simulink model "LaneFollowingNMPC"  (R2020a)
settings: Solver=FixedStepAuto  StartTime=0.0  StopTime=Duration  FixedStep=0.1  RelTol=1e-3  EnableMultiTasking=on
PreLoadFcn:
  | LaneFollowingUsingNMPCData
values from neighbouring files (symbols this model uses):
  Cf = 19000    [LaneFollowingStateFcn.m]    (also in LaneFollowingUsingNMPCData.m)
  Cr = 33000    [LaneFollowingStateFcn.m]    (also in LaneFollowingUsingNMPCData.m)
  Iz = 2875    [LaneFollowingStateFcn.m]    (also in LaneFollowingUsingNMPCData.m)
  lf = 1.2    [LaneFollowingStateFcn.m]    (also in LaneFollowingUsingNMPCData.m)
  lr = 1.6    [LaneFollowingStateFcn.m]    (also in LaneFollowingUsingNMPCData.m)
  m = 1575    [LaneFollowingStateFcn.m]    (also in LaneFollowingUsingNMPCData.m)
  rho = LaneFollowingGetCurvature(v_set,t)    [LaneFollowingUsingNMPCData.m]
  tau = 0.2    [LaneFollowingStateFcn.m]    (also in LaneFollowingUsingNMPCData.m)
  Ts = u(5)    [LaneFollowingEKFStateFcn.m]    (also in LaneFollowingUsingNMPCData.m = 0.1)
  v0 = 15    [LaneFollowingUsingNMPCData.m]
  v_set = 20    [LaneFollowingUsingNMPCData.m]
libraries: sharedTrackingLibrary x1, mpclib x1

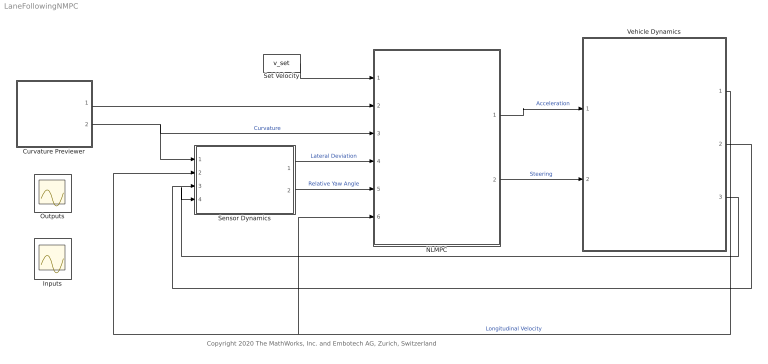
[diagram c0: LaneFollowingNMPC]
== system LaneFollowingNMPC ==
  note: Copyright 2020 The MathWorks, Inc. and Embotech AG, Zurich, Switzerland
  Curvature Previewer : Subsystem  mask{signal=rho, ts=Ts, steps=10}
      mask prompts: signal "Signal name"; ts "Sampling time"; steps "Number of previewing steps"
      mask init:
      | ts = evalin('base',get_param(gcbh,'ts'));
      | signal = evalin('base',get_param(gcbh,'signal'));
      | steps = evalin('base',get_param(gcbh,'steps'));
      | data = mpc_previewer_maskinit(signal,ts);
  Inputs : Scope
  NLMPC : Subsystem  VariantControl=controller_type ==1
  Outputs : Scope
  Sensor Dynamics : Subsystem
  Set Velocity : Constant  Value=v_set
  Vehicle Dynamics : Subsystem
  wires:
  Curvature Previewer/2(current) -> NLMPC/3(Current Curvature), Sensor Dynamics/1(Current curvature)  "Curvature"
  Vehicle Dynamics/2(Lateral Velocity) -> Sensor Dynamics/3(Lateral velocity)
  Vehicle Dynamics/3(Yaw Rate) -> Sensor Dynamics/4(Yaw rate)
  Vehicle Dynamics/1(Longitudinal Velocity) -> NLMPC/6(Longitudinal Velocity), Sensor Dynamics/2(Longitudinal velocity)  "Longitudinal Velocity"
  Curvature Previewer/1(sequence) -> NLMPC/2(Curvature Sequence)
  Sensor Dynamics/1(Lateral deviation) -> NLMPC/4(Lateral Deviation)  "Lateral Deviation"
  Sensor Dynamics/2(Relative yaw angle) -> NLMPC/5(Relative Yaw Angle)  "Relative Yaw Angle"
  Set Velocity/1 -> NLMPC/1(Set velocity)
  NLMPC/1(Acceleration) -> Vehicle Dynamics/1(Acceleration)  "Acceleration"
  NLMPC/2(Steering) -> Vehicle Dynamics/2(Steering)  "Steering"

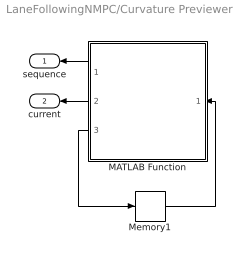
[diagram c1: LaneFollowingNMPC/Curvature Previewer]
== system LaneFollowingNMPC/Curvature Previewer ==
  MATLAB Function : MATLAB Function  TreatAsAtomicUnit=on
  Memory1 : Memory  InheritSampleTime=on  LinearizeAsDelay=on
  sequence : Outport  VectorParamsAs1DForOutWhenUnconnected=off
  current : Outport  Port=2  VectorParamsAs1DForOutWhenUnconnected=off
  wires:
  MATLAB Function/1(seq) -> sequence/1
  MATLAB Function/2(first) -> current/1
  Memory1/1 -> MATLAB Function/1(t)
  MATLAB Function/3(next_t) -> Memory1/1

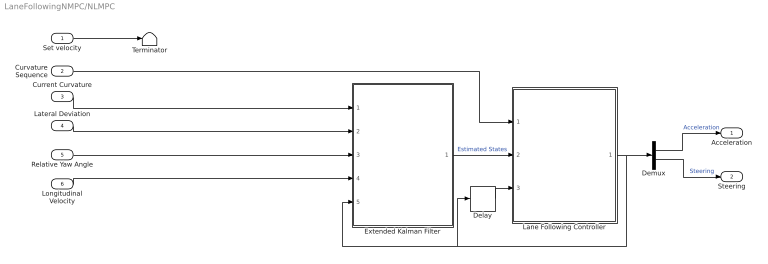
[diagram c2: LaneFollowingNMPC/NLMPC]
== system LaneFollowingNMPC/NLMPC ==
  Set velocity : Inport
  Curvature Sequence : Inport  Port=2
  Current Curvature : Inport  Port=3
  Lateral Deviation : Inport  Port=4
  Relative Yaw Angle : Inport  Port=5
  Longitudinal Velocity : Inport  Port=6
  Delay : Delay  DelayLength=1  InitialCondition=[0.2 0.3]
  Demux : Demux  Outputs=2
  Extended Kalman Filter : Subsystem
  Lane Following Controller : Subsystem
  Terminator : Terminator
  Acceleration : Outport  VectorParamsAs1DForOutWhenUnconnected=off
  Steering : Outport  Port=2  VectorParamsAs1DForOutWhenUnconnected=off
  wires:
  Extended Kalman Filter/1(xhat) -> Lane Following Controller/2(Estimated States)  "Estimated States"
  Lane Following Controller/1(Current MVs) -> Demux/1, Extended Kalman Filter/5(MVs), Delay/1
  Lateral Deviation/1 -> Extended Kalman Filter/2(Lateral Deviation)
  Curvature Sequence/1 -> Lane Following Controller/1(Curvature Sequence)
  Longitudinal Velocity/1 -> Extended Kalman Filter/4(Longitudinal Velocity)
  Delay/1 -> Lane Following Controller/3(Previous MVs)
  Relative Yaw Angle/1 -> Extended Kalman Filter/3(Relative Yaw Angle)
  Current Curvature/1 -> Extended Kalman Filter/1(Current Curvature)
  Set velocity/1 -> Terminator/1
  Demux/2 -> Steering/1  "Steering"
  Demux/1 -> Acceleration/1  "Acceleration"

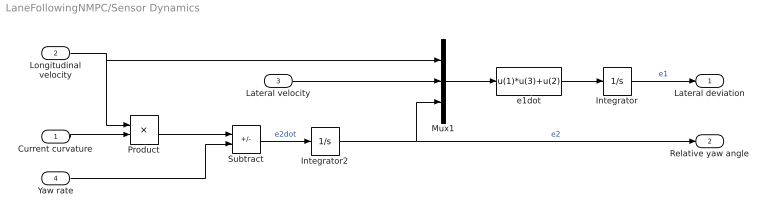
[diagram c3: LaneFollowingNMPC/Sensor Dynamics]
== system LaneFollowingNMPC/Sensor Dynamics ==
  Current curvature : Inport
  Longitudinal velocity : Inport  Port=2
  Lateral velocity : Inport  Port=3
  Yaw rate : Inport  Port=4
  Integrator : Integrator
  Integrator2 : Integrator
  Mux1 : Mux  Inputs=[1 1 1]
  Product : Product
  Subtract : Sum  Inputs=-+
  e1dot : Fcn  Expr=u(1)*u(3)+u(2)
  Lateral deviation : Outport  VectorParamsAs1DForOutWhenUnconnected=off
  Relative yaw angle : Outport  Port=2  VectorParamsAs1DForOutWhenUnconnected=off
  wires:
  Current curvature/1 -> Product/2
  Mux1/1 -> e1dot/1
  e1dot/1 -> Integrator/1
  Longitudinal velocity/1 -> Product/1, Mux1/1
  Lateral velocity/1 -> Mux1/2
  Integrator/1 -> Lateral deviation/1  "e1"
  Product/1 -> Subtract/1
  Yaw rate/1 -> Subtract/2
  Subtract/1 -> Integrator2/1  "e2dot"
  Integrator2/1 -> Mux1/3, Relative yaw angle/1  "e2"

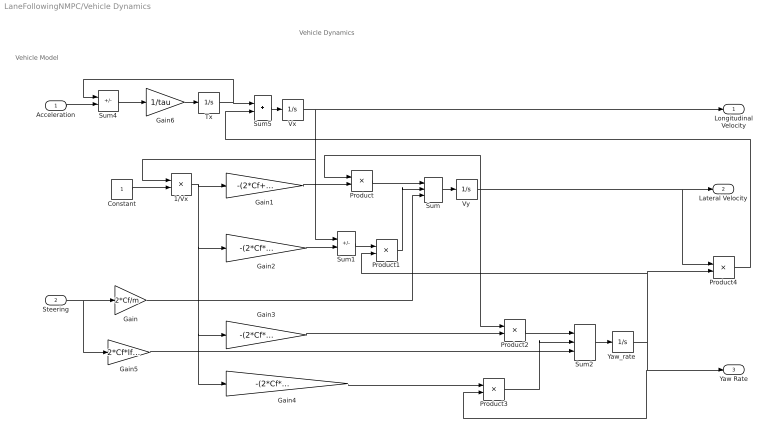
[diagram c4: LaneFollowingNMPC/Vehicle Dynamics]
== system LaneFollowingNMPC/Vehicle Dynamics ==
  note: Vehicle Model
  note: Vehicle Dynamics
  Acceleration : Inport
  Steering : Inport  Port=2
  1/Vx : Product  Inputs=/*
  Constant : Constant
  Gain : Gain  Gain=2*Cf/m
  Gain1 : Gain  Gain=-(2*Cf+2*Cr)/m
  Gain2 : Gain  Gain=-(2*Cf*lf-2*Cr*lr)/m
  Gain3 : Gain  Gain=-(2*Cf*lf-2*Cr*lr)/Iz
  Gain4 : Gain  Gain=-(2*Cf*lf^2+2*Cr*lr^2)/Iz
  Gain5 : Gain  Gain=2*Cf*lf/Iz
  Gain6 : Gain  Gain=1/tau
  Product{,1..4} (5 alike) : Product
  Sum : Sum  Inputs=+++
  Sum1 : Sum  Inputs=-+
  Sum2 : Sum  Inputs=+++
  Sum4 : Sum  Inputs=-+
  Sum5 : Sum
  Tx : Integrator
  Vx : Integrator  InitialCondition=v0
  Vy : Integrator
  "Yaw_rate " : Integrator
  Longitudinal Velocity : Outport  VectorParamsAs1DForOutWhenUnconnected=off
  Lateral Velocity : Outport  Port=2  VectorParamsAs1DForOutWhenUnconnected=off
  Yaw Rate : Outport  Port=3  VectorParamsAs1DForOutWhenUnconnected=off
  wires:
  Gain6/1 -> Tx/1
  Sum2/1 -> "Yaw_rate "/1
  Sum5/1 -> Vx/1
  Gain2/1 -> Sum1/2
  Gain4/1 -> Product3/1
  Constant/1 -> 1/Vx/2
  Gain3/1 -> Product2/2
  1/Vx/1 -> Gain4/1, Gain3/1, Gain2/1, Gain1/1
  Product2/1 -> Sum2/1
  Sum4/1 -> Gain6/1
  Acceleration/1 -> Sum4/2
  Tx/1 -> Sum5/1, Sum4/1
  Product3/1 -> Sum2/2
  Gain5/1 -> Sum2/3
  Product4/1 -> Sum5/2
  Sum1/1 -> Product1/1
  "Yaw_rate "/1 -> Yaw Rate/1, Product3/2, Product4/2, Product1/2
  Gain/1 -> Sum/3
  Steering/1 -> Gain/1, Gain5/1
  Gain1/1 -> Product/2
  Product/1 -> Sum/1
  Vy/1 -> Product/1, Lateral Velocity/1, Product4/1, Product2/1
  Sum/1 -> Vy/1
  Vx/1 -> Longitudinal Velocity/1, 1/Vx/1, Sum1/1
  Product1/1 -> Sum/2

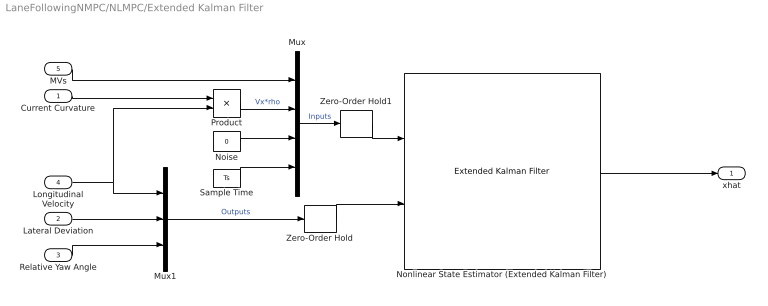
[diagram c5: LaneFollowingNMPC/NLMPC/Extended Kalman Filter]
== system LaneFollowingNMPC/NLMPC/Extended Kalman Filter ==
  Current Curvature : Inport
  Lateral Deviation : Inport  Port=2
  Relative Yaw Angle : Inport  Port=3
  Longitudinal Velocity : Inport  Port=4
  MVs : Inport  Port=5
  Mux : Mux
  Mux1 : Mux  Inputs=3
  Noise : Constant  Value=0
  Nonlinear State Estimator (Extended Kalman Filter) : sharedTrackingLibrary/Extended Kalman Filter  StateTransitionFcn=LaneFollowingEKFStateFcn  HasStateTransitionJacobianFcn=off  HasAdditiveProcessNoise=Additive  ProcessNoise=1e-4*eye(7)  HasTimeVaryingProcessNoise=off  HasStateTransitionFcnExtraArgument=1  InitialState=[0 0 v0 0 0 0 0]'  InitialStateCovariance=1e-4*eye(7)  MeasurementFcn1=LaneFollowingEKFMeasFcn  HasMeasurementJacobianFcn1=off  HasMeasurementEnablePort1=off  HasAdditiveMeasurementNoise1=Additive  MeasurementNoise1=1e-4*eye(3)  HasTimeVaryingMeasurementNoise1=off  HasMeasurementFcnExtraArgument1=0  MeasurementFcn2=myMeasurementFcn  HasMeasurementJacobianFcn2=off  HasMeasurementEnablePort2=off  HasAdditiveMeasurementNoise2=Additive  MeasurementNoise2=1  HasTimeVaryingMeasurementNoise2=off  HasMeasurementFcnExtraArgument2=0  MeasurementFcn3=myMeasurementFcn  HasMeasurementJacobianFcn3=off  HasMeasurementEnablePort3=off  HasAdditiveMeasurementNoise3=Additive  MeasurementNoise3=1  HasTimeVaryingMeasurementNoise3=off  HasMeasurementFcnExtraArgument3=0  MeasurementFcn4=myMeasurementFcn  HasMeasurementJacobianFcn4=off  HasMeasurementEnablePort4=off  HasAdditiveMeasurementNoise4=Additive  MeasurementNoise4=1  HasTimeVaryingMeasurementNoise4=off  HasMeasurementFcnExtraArgument4=0  MeasurementFcn5=myMeasurementFcn  HasMeasurementJacobianFcn5=off  HasMeasurementEnablePort5=off  HasAdditiveMeasurementNoise5=Additive  MeasurementNoise5=1  HasTimeVaryingMeasurementNoise5=off  HasMeasurementFcnExtraArgument5=0  EnableMultirate=off  StateTransitionFcnSampleTime=1  MeasurementFcn1SampleTime=1  MeasurementFcn2SampleTime=1  MeasurementFcn3SampleTime=1  MeasurementFcn4SampleTime=1  MeasurementFcn5SampleTime=1  UseCurrentEstimator=on  OutputStateCovariance=off  DataType=double  SampleTime=Ts  NumberOfMeasurements=1
  Product : Product
  Sample Time : Constant  Value=Ts
  Zero-Order Hold : ZeroOrderHold  SampleTime=Ts
  Zero-Order Hold1 : ZeroOrderHold  SampleTime=Ts
  xhat : Outport  VectorParamsAs1DForOutWhenUnconnected=off
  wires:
  Noise/1 -> Mux/3
  Zero-Order Hold/1 -> Nonlinear State Estimator (Extended Kalman Filter)/2
  MVs/1 -> Mux/1
  Sample Time/1 -> Mux/4
  Nonlinear State Estimator (Extended Kalman Filter)/1 -> xhat/1
  Mux1/1 -> Zero-Order Hold/1  "Outputs"
  Lateral Deviation/1 -> Mux1/2
  Longitudinal Velocity/1 -> Mux1/1, Product/2
  Relative Yaw Angle/1 -> Mux1/3
  Current Curvature/1 -> Product/1
  Product/1 -> Mux/2  "Vx*rho"
  Mux/1 -> Zero-Order Hold1/1  "Inputs"
  Zero-Order Hold1/1 -> Nonlinear State Estimator (Extended Kalman Filter)/1

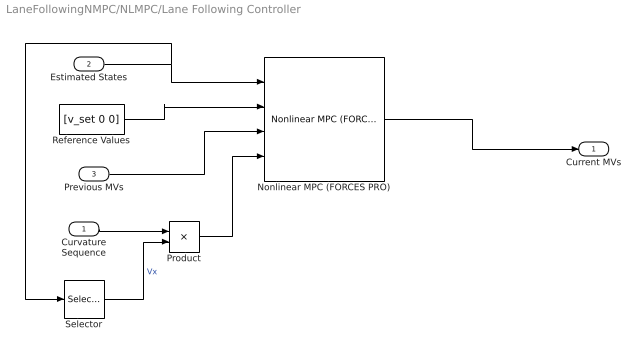
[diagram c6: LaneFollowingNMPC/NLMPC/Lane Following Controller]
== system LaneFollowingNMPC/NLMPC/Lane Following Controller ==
  Curvature Sequence : Inport
  Estimated States : Inport  Port=2
  Previous MVs : Inport  Port=3
  Nonlinear MPC (FORCES PRO) : mpclib/Nonlinear MPC (FORCES PRO)  SCDEnableBlockLinearizationSpecification=on  nlmpcobj=coredata  UseObjectTs=on  md_enabled=on  mvtarget_enabled=off  param_enabled=off  cost_enabled=off  mvseq_enabled=off  stateseq_enabled=off  ovseq_enabled=off  status_enabled=off  ov_min=off  ov_max=off  mv_min=off  mv_max=off  mvrate_min=off  mvrate_max=off  state_min=off  state_max=off  ov_weight=off  mv_weight=off  mvrate_weight=off  ecr_weight=off  nlp_initialize=off
  Product : Product
  Reference Values : Constant  Value=[v_set 0 0]  VectorParams1D=off
  Selector : Selector  InputPortWidth=7  IndexOptions=Index vector (dialog)  Indices=[3]  OutputSizes=1
  Current MVs : Outport  VectorParamsAs1DForOutWhenUnconnected=off
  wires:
  Estimated States/1 -> Nonlinear MPC (FORCES PRO)/1, Selector/1
  Selector/1 -> Product/2  "Vx"
  Curvature Sequence/1 -> Product/1
  Reference Values/1 -> Nonlinear MPC (FORCES PRO)/2
  Previous MVs/1 -> Nonlinear MPC (FORCES PRO)/3
  Product/1 -> Nonlinear MPC (FORCES PRO)/4
  Nonlinear MPC (FORCES PRO)/1 -> Current MVs/1

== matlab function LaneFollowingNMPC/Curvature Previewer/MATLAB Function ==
function [seq,first,next_t] = fcn(data,steps,t)
%#codegen
[seq,first,next_t] = mpcblock_preview('md',data,steps,t);
